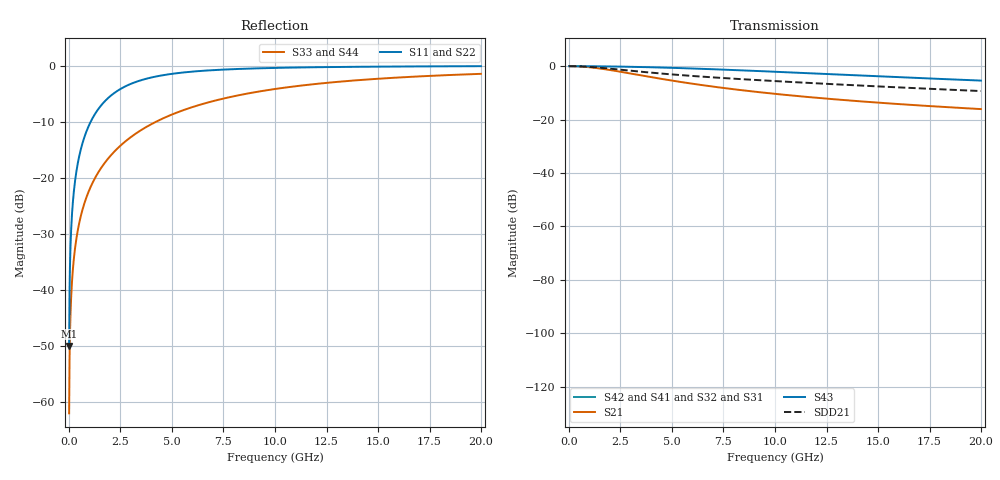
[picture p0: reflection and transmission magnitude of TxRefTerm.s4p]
! 2 pF port 1 to ground & 0.5 pF port 2 to ground  (Model #2 from T10/07-267r0)
! reasonably models 6G SAS high frequency limits for SDD22 & SCD22
!  Mike Jenkins  5 June 2007
# MHz S MA R 50
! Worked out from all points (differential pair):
!   1999 points, 10 MHz to 19.99 GHz, reference 50 ohm
!   strongest paths, dB at 10 MHz, 5 GHz, 10 GHz, 15 GHz, 19.99 GHz:
!     S43: 0.0, -0.6, -2.1, -3.8, -5.4
!     S21: 0.0, -5.4, -10.4, -13.7, -16.1
!     S42: -, -, -, -, -
!     S41: -, -, -, -, -
!     S32: -, -, -, -, -
!     S31: -, -, -, -, -
!   taken as a pair (ports 3,1 in; 4,2 out), SDD21 dB: 0.0, -3.1, -5.6, -7.6, -9.3
!   lowest |S11| = -50.1 dB at 10 MHz (marker M1), VSWR 1.01, Z = 50 - j0.314 ohm
!   |S11| at or under -10 dB: start of sweep to 1.061 GHz
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10  0.003142 -90.2  1 -0.2  0 0.0  0 0.0
    1 -0.2  0.003142 -90.2  0 0.0  0 0.0
    0 0.0  0 0.0  0.000785 -90.0  1 -0.0
    0 0.0  0 0.0  1 -0.0  0.000785 -90.0
200  0.06271 -93.6  0.998 -3.6  0 0.0  0 0.0
     0.998 -3.6  0.06271 -93.6  0 0.0  0 0.0
     0 0.0  0 0.0  0.01571 -90.9  0.9999 -0.9
     0 0.0  0 0.0  0.9999 -0.9  0.01571 -90.9
640  0.1971 -101.4  0.9804 -11.4  0 0.0  0 0.0
     0.9804 -11.4  0.1971 -101.4  0 0.0  0 0.0
     0 0.0  0 0.0  0.0502 -92.9  0.9987 -2.9
     0 0.0  0 0.0  0.9987 -2.9  0.0502 -92.9
1550  0.4378 -116.0  0.8991 -26.0  0 0.0  0 0.0
      0.8991 -26.0  0.4378 -116.0  0 0.0  0 0.0
      0 0.0  0 0.0  0.1208 -96.9  0.9927 -6.9
      0 0.0  0 0.0  0.9927 -6.9  0.1208 -96.9
3060  0.693 -133.9  0.7209 -43.9  0 0.0  0 0.0
      0.7209 -43.9  0.693 -133.9  0 0.0  0 0.0
      0 0.0  0 0.0  0.2337 -103.5  0.9723 -13.5
      0 0.0  0 0.0  0.9723 -13.5  0.2337 -103.5
8040  0.9298 -158.4  0.3681 -68.4  0 0.0  0 0.0
      0.3681 -68.4  0.9298 -158.4  0 0.0  0 0.0
      0 0.0  0 0.0  0.5339 -122.3  0.8455 -32.3
      0 0.0  0 0.0  0.8455 -32.3  0.5339 -122.3
19990  0.9876 -170.9  0.1573 -81.0  0 0.0  0 0.0
       0.1573 -81.0  0.9876 -170.9  0 0.0  0 0.0
       0 0.0  0 0.0  0.8434 -147.5  0.5372 -57.5
       0 0.0  0 0.0  0.5372 -57.5  0.8434 -147.5
